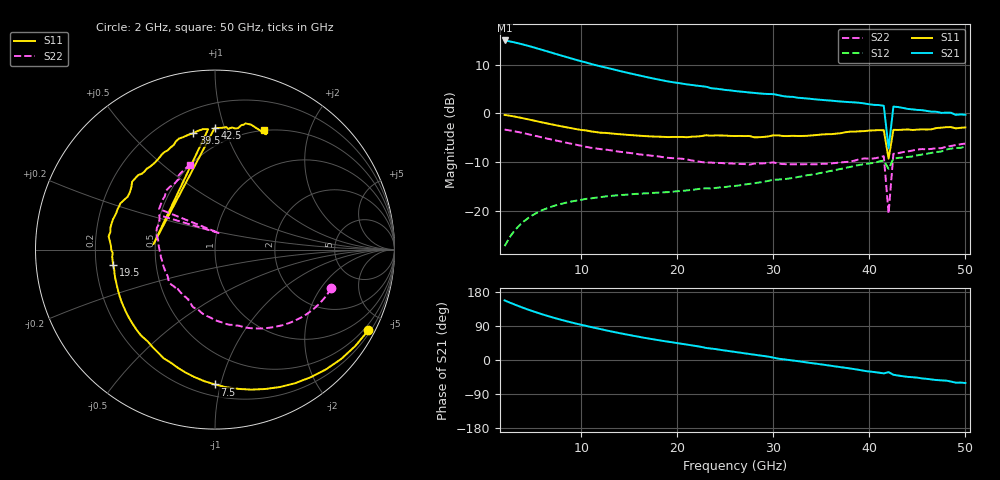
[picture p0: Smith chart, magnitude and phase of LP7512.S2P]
! Litton, dev L7512 #1 no C, Idss=40.1mA, Vds=2V, Vgs=-0.34, Ids=10.14mA
! 19-NOV-94 15:05
! SRITABLE TWO_PORT 97
# GHZ S RI R 50
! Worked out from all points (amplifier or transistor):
!   97 points, 2 GHz to 50 GHz, reference 50 ohm
!   highest |S21| = 15.0 dB at 2 GHz (marker M1)
!   |S21| within 3 dB of that: start of sweep to 7.743 GHz
!   unconditionally stable (mu >= 1): 41.55 GHz to 42.45 GHz
!   at 10 GHz: K = 0.53, MSG = 14.2 dB, |S12| = -17.7 dB
!   at 26 GHz: K = 0.94, MSG = 9.7 dB, |S12| = -14.9 dB
!   at 50 GHz: K = 0.65, MSG = 3.3 dB, |S12| = -6.8 dB
!   S11 on the Smith chart (normalised r, x): 2 GHz: 0.30, -4.03; 7.5 GHz: 0.28, -0.96; 19.5 GHz: 0.27, -0.07; 39.5 GHz: 0.34, +0.77; 42.5 GHz: 0.37, +0.93; 50 GHz: 0.50, +1.37
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2  0.8546 -0.4496  -5.157 2.163  0.0129 0.0417  0.6483 -0.2156
2.5  0.7825 -0.5363  -4.832 2.579  0.0193 0.0497  0.6185 -0.2596
3.5  0.6185 -0.6672  -4.096 3.219  0.0337 0.0621  0.5511 -0.3294
4.5  0.4462 -0.7445  -3.317 3.62  0.0491 0.0699  0.479 -0.379
6  0.2025 -0.7802  -2.223 3.858  0.0708 0.0746  0.3767 -0.4209
7.5  -0.0024 -0.7511  -1.297 3.808  0.0889 0.0739  0.2891 -0.4369
9  -0.1639 -0.6852  -0.5593 3.601  0.1042 0.0698  0.213 -0.4387
10  -0.2466 -0.6299  -0.1674 3.412  0.1122 0.0665  0.1697 -0.434
11.5  -0.3486 -0.5423  0.3129 3.106  0.1227 0.0608  0.1155 -0.4228
13.5  -0.4577 -0.4155  0.8044 2.68  0.1346 0.052  0.0473 -0.4097
15.5  -0.5203 -0.2919  1.125 2.252  0.1429 0.0439  -0.0099 -0.3887
18  -0.5562 -0.1576  1.357 1.765  0.1501 0.0358  -0.0697 -0.3562
19.5  -0.5678 -0.0845  1.44 1.518  0.1544 0.0333  -0.0964 -0.3347
23  -0.5928 0.0735  1.595 0.9888  0.1695 0.0238  -0.1478 -0.2763
26  -0.5483 0.2085  1.581 0.6139  0.1797 0.0201  -0.1931 -0.2371
30  -0.4617 0.378  1.567 0.1745  0.2089 0.013  -0.2554 -0.1845
34  -0.3176 0.5034  1.391 -0.202  0.2362 -0.0024  -0.293 -0.0702
39.5  -0.1212 0.648  1.108 -0.6083  0.2979 -0.0509  -0.3238 0.1221
41.5  -0.0382 0.6703  0.9765 -0.692  0.3199 -0.076  -0.3103 0.1914
42  -0.3424 0.0306  0.3702 -0.2318  0.2542 -0.0922  0.0254 0.091
42.5  -0.0013 0.6785  0.9125 -0.7384  0.3307 -0.0962  -0.3117 0.2265
50  0.2708 0.666  0.4746 -0.8459  0.3828 -0.253  -0.137 0.4722
